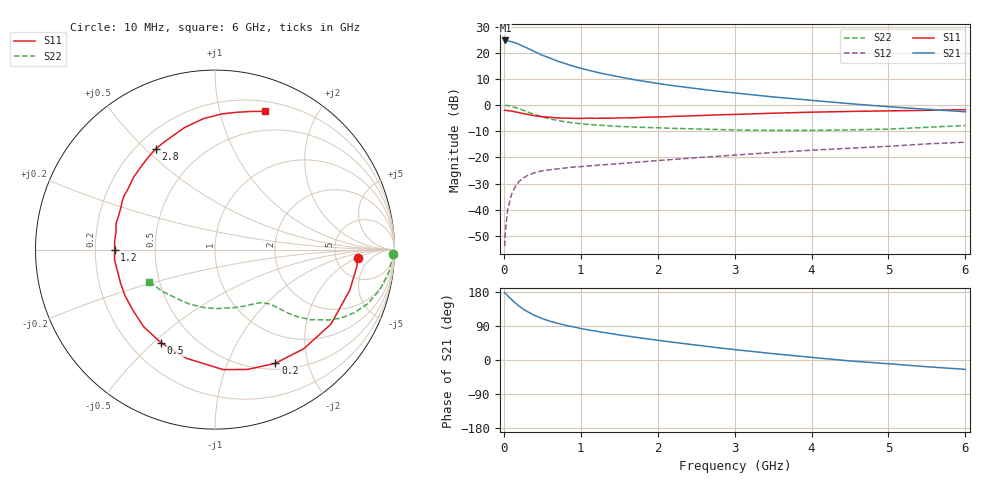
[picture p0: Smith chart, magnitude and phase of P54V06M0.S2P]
! SIEMENS Small Signal Semiconductors
! BFP183
! Si NPN RF Bipolar Junction Transistor in SOT143
! VCE = 4 V  IC = 6 mA
! Common Emitter S-Parameters:  March  1996
# GHz  S  MA  R  50
!  f  S11  S21  S12  S22
! GHz  MAG  ANG  MAG  ANG  MAG  ANG  MAG  ANG
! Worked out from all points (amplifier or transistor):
!   36 points, 10 MHz to 6 GHz, reference 50 ohm
!   highest |S21| = 24.7 dB at 20 MHz (marker M1)
!   |S21| within 3 dB of that: start of sweep to 310.6 MHz
!   unconditionally stable (mu >= 1): 1.484 GHz to 5.632 GHz
!   at 250 MHz: K = 0.23, MSG = 25.2 dB, |S12| = -28.0 dB
!   at 1.4 GHz: K = 0.98, MSG = 17.0 dB, |S12| = -22.6 dB
!   at 6 GHz: K = 0.94, MSG = 5.8 dB, |S12| = -14.2 dB
!   lowest NFmin = 1.20 dB at 450 MHz
!   S11 on the Smith chart (normalised r, x): 10 MHz: 8.31, -2.02; 200 MHz: 0.58, -1.51; 500 MHz: 0.33, -0.53; 1.2 GHz: 0.28, -0.00; 2.8 GHz: 0.28, +0.54; 6 GHz: 0.30, +1.38
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0.01  0.7961 -3.2  17.11 178.0  0.002 79.5  0.9922 -1.4
0.02  0.796 -6.8  17.26 176.1  0.0038 81.2  0.988 -2.9
0.05  0.7843 -16.7  16.98 169.5  0.0101 82.3  0.9779 -7.0
0.1  0.7682 -32.6  16.27 159.7  0.0195 72.7  0.9461 -13.6
0.15  0.7416 -48.1  15.5 150.3  0.0278 67.0  0.9021 -19.6
0.2  0.7171 -62.0  14.5 141.9  0.0347 60.4  0.8503 -24.5
0.25  0.6921 -74.7  13.37 134.6  0.04 55.4  0.7987 -28.6
0.3  0.6702 -86.1  12.44 128.5  0.0445 51.2  0.7456 -31.7
0.4  0.6265 -104.6  10.55 117.6  0.0509 45.0  0.6614 -36.2
0.5  0.6 -120.1  9.002 109.2  0.0555 40.2  0.5952 -39.0
0.6  0.5852 -132.9  7.918 102.4  0.0579 37.6  0.5455 -40.8
0.7  0.5688 -143.2  6.923 96.8  0.0604 35.9  0.5065 -41.9
0.9  0.5587 -160.0  5.591 87.5  0.0651 33.8  0.457 -43.6
1.1  0.5628 -174.2  4.656 79.3  0.0685 33.6  0.4262 -45.2
1.2  0.5591 -179.9  4.283 76.0  0.0703 33.1  0.4166 -46.1
1.7  0.574 156.1  3.054 60.4  0.0802 34.2  0.3801 -51.9
2.2  0.6073 138.2  2.358 46.8  0.0911 34.6  0.3589 -59.6
2.8  0.6512 120.5  1.839 32.0  0.1055 33.9  0.3413 -71.3
3.5  0.7005 104.1  1.435 16.7  0.1239 32.2  0.3291 -87.8
4.5  0.7573 87.0  1.065 -2.5  0.1497 27.1  0.336 -116.1
5.5  0.7952 75.4  0.833 -17.8  0.1813 21.7  0.3762 -142.2
6  0.8187 70.2  0.746 -24.7  0.1951 17.5  0.4074 -154.1
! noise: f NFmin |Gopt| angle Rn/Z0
0.45  1.2  0.21  41  0.24
0.9  1.25  0.24  101  0.21
1.8  2  0.32  175  0.14
